(* 	
	Program Name: 	ACS_READ_AXIS_VARIABLES
	Purpose:		(To be used only by Input Scan Function) Copy Drive Variables into shadow memory for program access 
*)
PROGRAM ACS_READ_AXIS_VARIABLES
VAR_IN_OUT
	Axis:ACS_DRIVE_TYPE;
END_VAR

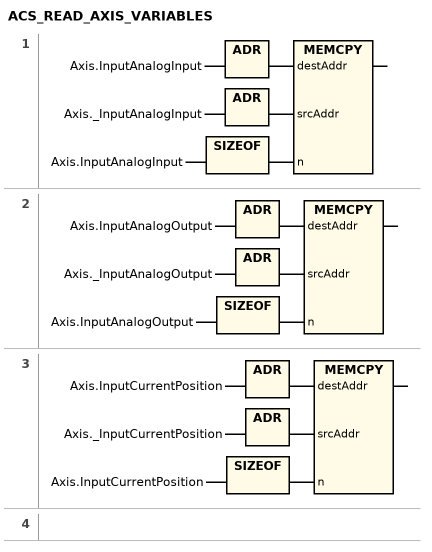
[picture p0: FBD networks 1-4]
// NETWORK 1
MEMCPY(destAddr := ADR(Axis.InputAnalogInput), srcAddr := ADR(Axis._InputAnalogInput), n := SIZEOF(Axis.InputAnalogInput));

// NETWORK 2
MEMCPY(destAddr := ADR(Axis.InputAnalogOutput), srcAddr := ADR(Axis._InputAnalogOutput), n := SIZEOF(Axis.InputAnalogOutput));

// NETWORK 3
MEMCPY(destAddr := ADR(Axis.InputCurrentPosition), srcAddr := ADR(Axis._InputCurrentPosition), n := SIZEOF(Axis.InputCurrentPosition));

// NETWORK 4

END_PROGRAM
